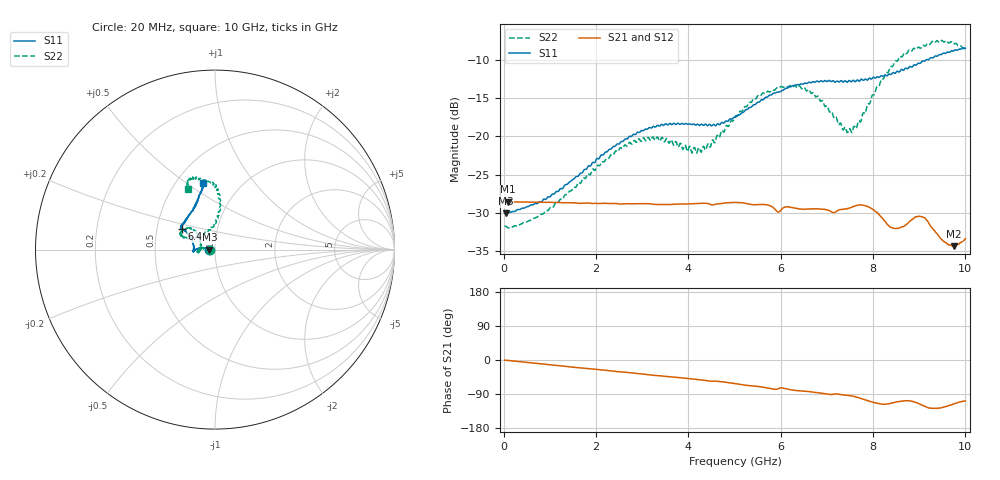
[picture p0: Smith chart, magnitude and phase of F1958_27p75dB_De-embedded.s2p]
! Integrated Device Technology
! Corporate Headquarters
! 6024 Silver Creek Valley Road
! San Jose, CA 95138  USA
! Phone:  1-408-284-8200
! Toll Free:  1-800-223-1366
! Webpage:  http://www.idt.com/
! Timing and RF Division
! 515 Groton Road, Suite 102
! Westford, MA 01886-6024
! Device:  F1958
! Description: 7-bit 0.25 dB Digital Step Attenuator
! Frequency:  0.001 -  6.000 GHz
! Package:  4x4 mm Thin QFN Plastic Package: 24 pin
! Ports:  2 RF, 12 DC
!  Pin  1  = D0
!  Pin  2  = VDD
!  Pin  3  = VMODE
!  Pin  4  = GND
!  Pin  5  = RF1  =  Port 1
!  Pin  6  = GND
!  Pin  7  = GND
!  Pin  8  = GND
!  Pin  9  = GND
!  Pin 10  = GND
!  Pin 11  = GND
!  Pin 12  = GND
!  Pin 13  = GND
!  Pin 14  = RF2  =  Port 2
!  Pin 15  = GND
!  Pin 16  = LE
!  Pin 17  = CLK
!  Pin 18  = DATA
!  Pin 19  = D6
!  Pin 20  = D5
!  Pin 21  = D4
!  Pin 22  = D3
!  Pin 23  = D2
!  Pin 24  = D1
! State:  111
! Atten State:  27.75 dB
! Voltage:  +3.30 Volts
! Current:  0.258 mA
! Data:  The device was measured on a F1958 evaluation board which has
!  individual transmission lines to the RF pins.  Data was collected
!  using a calibrated network analyzer.  The evaluation board was
!  de-embedded using Automatic Fixture Removal (AFR).
!  The reference plane is the edge of the package pin.
! Misc:
!  Action Tracker AT0419
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# GHz S dB R 50
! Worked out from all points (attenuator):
!   500 points, 20 MHz to 10 GHz, reference 50 ohm
!   highest |S21| = -28.54 dB at 100 MHz (marker M1); lowest = -34.3 dB at 9.76 GHz (marker M2)
!   lowest |S11| = -30.0 dB at 40 MHz (marker M3), VSWR 1.07, Z = 46.9 - j0.0449 ohm
!   |S11| at or under -10 dB: start of sweep to 9.151 GHz
!   |S22| runs from -31.9 to -7.5 dB; largest |S21 - S12| = 0.00024
!   S11 on the Smith chart (normalised r, x): 20 MHz: 0.94, -0.00; 6.4 GHz: 0.67, +0.16; 10 GHz: 0.68, +0.58
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0.02  -29.99 -178.9  -28.55 -0.3  -28.55 -0.2  -31.73 -178.9
0.04  -30.02 -179.1  -28.55 -0.4  -28.54 -0.4  -31.71 -178.5
0.1  -29.91 179.3  -28.54 -1.2  -28.54 -1.2  -31.95 179.9
0.84  -28.40 170.8  -28.60 -10.6  -28.59 -10.6  -30.15 172.2
1.7  -24.76 170.6  -28.72 -21.0  -28.72 -21.0  -25.67 171.1
2.62  -20.38 176.6  -28.80 -32.1  -28.78 -32.2  -21.11 -180.0
3.36  -18.63 -176.0  -28.88 -41.5  -28.88 -41.6  -20.43 -170.0
4.24  -18.57 -179.4  -28.74 -52.0  -28.76 -52.1  -21.52 168.2
5.02  -17.50 160.4  -28.61 -62.4  -28.63 -62.5  -17.32 137.8
5.58  -15.23 150.3  -28.90 -71.0  -28.91 -71.0  -14.60 139.5
5.94  -14.19 148.1  -29.86 -76.0  -29.87 -75.9  -13.69 148.3
6.4  -13.26 147.7  -29.47 -81.3  -29.48 -81.2  -13.41 155.4
6.68  -12.90 146.6  -29.46 -84.3  -29.48 -84.2  -14.35 157.4
7.5  -12.74 138.3  -29.33 -94.0  -29.34 -93.9  -18.97 119.3
7.68  -12.70 135.4  -28.96 -99.1  -28.96 -99.1  -18.00 99.1
7.9  -12.51 128.9  -29.19 -107.8  -29.18 -107.9  -15.71 88.9
8.34  -11.87 118.9  -31.63 -115.6  -31.65 -115.8  -11.49 83.7
8.66  -11.37 113.2  -31.75 -107.8  -31.75 -107.8  -9.26 87.5
9.06  -10.21 106.8  -30.49 -118.9  -30.55 -119.0  -8.26 97.3
9.52  -9.12 101.7  -33.67 -124.5  -33.66 -124.7  -7.62 109.1
9.76  -8.78 100.2  -34.33 -115.3  -34.27 -115.5  -7.92 111.3
10  -8.49 100.0  -33.36 -108.3  -33.33 -108.5  -8.62 113.7
